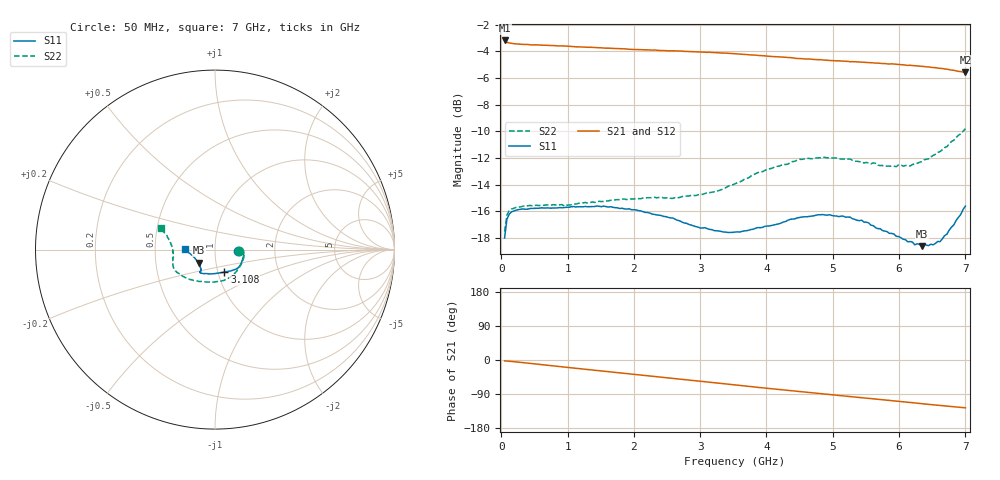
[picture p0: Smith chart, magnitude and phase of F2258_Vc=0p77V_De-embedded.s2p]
! Integrated Device Technology
! Corporate Headquarters
! 6024 Silver Creek Valley Road
! San Jose, CA 95138  USA
! Phone:  1-408-284-8200
! Toll Free:  1-800-223-1366
! Webpage:  http://www.idt.com/
! Timing and RF Division
! 515 Groton Road, Suite 102
! Westford, MA 01886-6024
! Device:  F2258
! Description: Voltage Variable RF Attenuator
! Frequency:  50.0 -  6000.00 MHz
! Package:  3x3 mm Thin QFN Plastic Package: 16 pin
! Ports:  2 RF, 2 DC
!  Pin  1  = NC
!  Pin  2  = NC
!  Pin  3  = RF2  = Port 2
!  Pin  4  = GND
!  Pin  5  = Vdd
!  Pin  6  = NC
!  Pin  7  = VCTRL
!  Pin  8  = NC
!  Pin  9  = GND
!  Pin 10  = RF1  = Port 1
!  Pin 11  = NC
!  Pin 12  = NC
!  Pin 13  = NC
!  Pin 14  = NC
!  Pin 15  = NC
!  Pin 16  = NC
! Vcntrl:  0.770 Volts
! Vdd:  +3.300 Volts
! Current:  1.130 mA
! Data:  The device was measured on a the F2258 evaluation board which has
!  individual transmission lines to the RF pins.  Data was collected
!  using a calibrated network analyzer.  The evaluation board was
!  de-embedded using a TRL calibration technique.
!  The reference plane is the edge of the package pin.
! Misc:  SN 10
!  Action Tracker AT0285
! Date Measured:  2014-12-10
! Date:  2016-01-13  MJV
! Note:
!  Integrated Device Technology supplies this data as a sample of measured
!  data at the package pin for this product.  Your particular data for this
!  product may vary.
!  Data was taken at 25 degrees C.
!  Integrated Device Technology reserves the right to change this data at anytime.
!Freq_(GHz)  S11M_(dB)  S11P_(deg)  S21M_(dB)  S21P_(deg)  S12M_(dB)  S12P_(deg)  S22M_(dB)  S22P_(deg)
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# GHz S dB R 50
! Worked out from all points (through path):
!   201 points, 50 MHz to 7 GHz, reference 50 ohm
!   highest |S21| = -3.19 dB at 50 MHz (marker M1); lowest = -5.6 dB at 7 GHz (marker M2)
!   group delay of S21, straight-line fit = 49.9 ps
!   lowest |S11| = -18.6 dB at 6.34 GHz (marker M3), VSWR 1.27, Z = 41.2 - j6.12 ohm
!   |S11| at or under -10 dB: start of sweep to end of sweep
!   |S22| runs from -17.5 to -9.8 dB; largest |S21 - S12| = 0.0027
!   S11 on the Smith chart (normalised r, x): 50 MHz: 1.29, -0.02; 3.108 GHz: 1.07, -0.28; 7 GHz: 0.72, +0.00
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0.05  -18.00 -2.8  -3.19 -2.3  -3.21 -2.3  -17.54 -3.3
0.08475  -16.60 -2.9  -3.34 -2.7  -3.34 -2.7  -16.28 -3.9
0.15425  -16.04 -4.1  -3.41 -3.8  -3.42 -3.8  -15.82 -6.4
0.6755  -15.75 -17.0  -3.56 -13.5  -3.57 -13.5  -15.53 -25.0
0.9535  -15.71 -24.8  -3.61 -18.7  -3.61 -18.7  -15.63 -35.9
1.2315  -15.67 -30.2  -3.69 -23.8  -3.70 -23.8  -15.37 -45.1
1.6485  -15.66 -37.2  -3.78 -31.4  -3.80 -31.4  -15.18 -57.5
2.37825  -16.29 -47.8  -3.94 -44.5  -3.95 -44.5  -14.97 -77.4
2.58675  -16.50 -52.2  -3.98 -48.3  -3.97 -48.3  -15.04 -83.8
3.108  -17.31 -67.3  -4.09 -57.9  -4.08 -57.9  -14.61 -102.8
3.525  -17.56 -84.5  -4.19 -65.8  -4.19 -65.8  -13.95 -119.5
4.0115  -17.11 -104.6  -4.38 -74.8  -4.38 -74.8  -12.85 -136.7
4.498  -16.47 -117.8  -4.55 -83.5  -4.58 -83.5  -12.11 -149.4
4.7065  -16.35 -120.1  -4.62 -87.1  -4.63 -87.1  -12.05 -153.7
5.2625  -16.45 -123.9  -4.79 -96.6  -4.80 -96.6  -12.09 -162.9
5.5405  -16.87 -124.2  -4.86 -101.3  -4.87 -101.3  -12.38 -167.7
5.85325  -17.66 -126.7  -4.96 -106.6  -4.95 -106.7  -12.62 -174.2
6.166  -18.27 -133.5  -5.06 -112.1  -5.06 -112.1  -12.60 178.7
6.33975  -18.62 -141.3  -5.13 -115.1  -5.13 -115.2  -12.28 173.9
6.61775  -18.28 -159.2  -5.28 -119.9  -5.29 -119.9  -11.52 166.8
6.82625  -17.01 -171.1  -5.43 -123.5  -5.43 -123.5  -10.67 162.1
7  -15.61 179.5  -5.58 -126.3  -5.59 -126.3  -9.81 158.5
